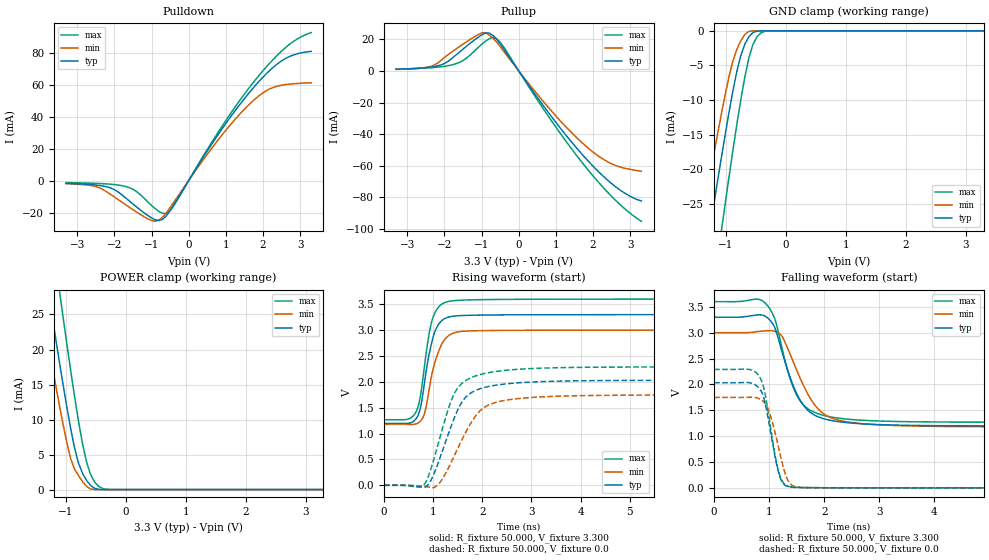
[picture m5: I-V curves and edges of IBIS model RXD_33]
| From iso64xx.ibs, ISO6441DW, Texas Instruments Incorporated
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|   RXD_33 Model
[Model]   RXD_33
Model_type   3-state
| Signals   RXD
Vmeas = 2.2V   |Reference voltage for timing measurements
Cref = 15pF   |Timing specification test load capacitance value
Vref = 0   |Timing specification test load voltage; GND
| variable   typ   min   max
C_comp   2.1pF   1.7pF   2.5pF
|   typ   min   max
[Temperature Range]   25.0   -40   125
[Voltage range]   3.3V   3.0V   3.6V
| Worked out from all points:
|   slope of the pulldown table from 0 to 0.495 V, typ, clamps not added: 27 ohm
|   slope of the pullup table from 0 to 0.495 V, typ, clamps not added: 29.8 ohm
|   GND clamp passes 1 mA (typ) near -0.63 V on its own axis
|   POWER clamp passes 1 mA (typ) near -0.62 V on its own axis
|   rising waveform, R_fixture 50.000, V_fixture 3.300: 20-80 % time 238ps typ, 270ps min, 219ps max; typ from 1.2 V to 3.3 V
|   rising waveform, R_fixture 50.000, V_fixture 0.0: 20-80 % time 505ps typ, 594ps min, 466ps max; typ from 0 V to 2.03 V
|   falling waveform, R_fixture 50.000, V_fixture 3.300: 20-80 % time 442ps typ, 514ps min, 392ps max; typ from 3.3 V to 1.2 V
|   falling waveform, R_fixture 50.000, V_fixture 0.0: 20-80 % time 217ps typ, 247ps min, 215ps max; typ from 2.03 V to 0 V
[Pulldown]
|Voltage   I(typ)   I(min)   I(max)
-3.3V     -1.746mA   -1.954mA   -1.317mA
-2.4V     -3.065mA   -4.531mA   -1.845mA
-1.7V     -10.79mA   -15.08mA   -3.688mA
-1.4V     -16.56mA   -19.75mA   -6.913mA
-900mV    -24.57mA   -25.5mA    -17.6mA
-600mV    -22.05mA   -20.21mA   -20.59mA
-400mV    -15.17mA   -13.54mA   -15.73mA
700mV     25.56mA    22.64mA    26.86mA
1.7V      56.99mA    49.23mA    60.23mA
2.1V      67.13mA    56.39mA    71.43mA
2.5V      74.94mA    59.69mA    81.03mA
3.3V      80.92mA    61.24mA    92.67mA
[Pullup]
|Voltage   I(typ)   I(min)   I(max)
-3.3V     1.146mA    992.8uA    1.173mA
-2.5V     2.119mA    2.237mA    1.881mA
-2.1V     3.82mA     6.606mA    2.666mA
-1.5V     13.89mA    17.02mA    6.669mA
-1V       22.84mA    24.1mA     16.9mA
-800mV    24.1mA     22.86mA    20.41mA
-600mV    20.3mA     18.51mA    20.5mA
-400mV    13.92mA    12.34mA    14.99mA
700mV     -23.25mA   -20.4mA    -25.37mA
1.7V      -52.69mA   -45.38mA   -57.86mA
2.5V      -71.39mA   -58.82mA   -79.5mA
3.3V      -82.38mA   -63.55mA   -95.26mA
[GND_clamp]
|Voltage   I(typ)   I(min)   I(max)
-3.3V     -145mA     -121.7mA   -175mA
-1.424V   -37.25mA   -28.36mA   -50.84mA
-1.29V    -29.79mA   -21.9mA    -42.24mA
-1.223V   -26.11mA   -18.72mA   -37.97mA
-1.089V   -18.87mA   -12.5mA    -29.55mA
-1.022V   -15.36mA   -9.534mA   -25.41mA
-821mV    -5.911mA   -2.691mA   -13.56mA
-754mV    -3.587mA   -1.433mA   -9.951mA
-620mV    -866.1uA   -93.64uA   -3.947mA
-486mV    -44.39uA   -245.8nA   -879.4uA
-352mV    -377.3nA   -292.5pA   -83.51uA
3.3V      0A         0A         0A
[POWER_clamp]
|Voltage   I(typ)   I(min)   I(max)
-3.3V     144.8mA    121.5mA    175.1mA
-1.457V   37.64mA    28.8mA     50.97mA
-1.39V    33.85mA    25.52mA    46.59mA
-1.256V   26.35mA    19.04mA    37.91mA
-1.122V   19.03mA    12.73mA    29.39mA
-1.055V   15.47mA    9.712mA    25.21mA
-921mV    8.813mA    4.477mA    17.12mA
-854mV    5.956mA    2.907mA    13.29mA
-720mV    2.301mA    1.133mA    6.51mA
-586mV    594.1uA    80.22uA    2.141mA
-318mV    345.9nA    220.3pA    41.12uA
3.3V      0A         0A         0A
[Ramp]
| variable   typ   min   max
dV/dt_r   1.219/0.505n   1.049/0.594n   1.374/0.467n
dV/dt_f   1.262/0.442n   1.093/0.514n   1.399/0.392n
R_load = 50.000
[Rising Waveform]
R_fixture= 50.000
V_fixture= 3.300
V_fixture_min= 3.000
V_fixture_max= 3.600
|time   V(typ)   V(min)   V(max)
0s        1.197V     1.178V     1.268V
469ps     1.196V     1.177V     1.274V
644ps     1.274V     1.185V     1.404V
733ps     1.462V     1.231V     1.675V
824ps     1.976V     1.388V     2.299V
913ps     2.502V     1.815V     2.896V
981ps     2.793V     2.169V     3.196V
1.17ns    3.178V     2.717V     3.499V
1.341ns   3.259V     2.911V     3.56V
15ns      3.3V       3V         3.6V
[Rising Waveform]
R_fixture= 50.000
V_fixture= 0.0
V_fixture_min= 0.0
V_fixture_max= 0.0
|time   V(typ)   V(min)   V(max)
0s        385.3nV    211.2nV    1.176uV
820ps     -34.98mV   -20.2mV    18.14mV
933ps     57.96mV    -40.03mV   254mV
1.105ns   437.4mV    19.91mV    808.4mV
1.454ns   1.354V     617.7mV    1.812V
1.634ns   1.672V     969.8mV    2.006V
1.864ns   1.834V     1.34V      2.115V
2.204ns   1.925V     1.581V     2.191V
4.104ns   2.023V     1.735V     2.282V
15ns      2.031V     1.748V     2.289V
[Falling Waveform]
R_fixture= 50.000
V_fixture= 3.300
V_fixture_min= 3.000
V_fixture_max= 3.600
|time   V(typ)   V(min)   V(max)
0s        3.3V       3V         3.6V
914ps     3.326V     3.033V     3.586V
1.105ns   3.091V     3.027V     3.26V
1.237ns   2.618V     2.927V     2.689V
1.388ns   2.113V     2.565V     2.084V
1.538ns   1.743V     2.18V      1.722V
1.864ns   1.385V     1.555V     1.442V
2.244ns   1.282V     1.314V     1.35V
4.338ns   1.201V     1.185V     1.272V
15ns      1.197V     1.178V     1.268V
[Falling Waveform]
R_fixture= 50.000
V_fixture= 0.0
V_fixture_min= 0.0
V_fixture_max= 0.0
|time   V(typ)   V(min)   V(max)
0s        2.031V     1.748V     2.289V
605ps     2.036V     1.75V      2.294V
817ps     1.927V     1.725V     2.162V
899ps     1.75V      1.664V     1.95V
986ps     1.321V     1.514V     1.442V
1.102ns   633.7mV    1.091V     661.1mV
1.172ns   292.6mV    774.7mV    312mV
1.294ns   47.58mV    266.2mV    59.06mV
1.404ns   13.21mV    60.12mV    17.7mV
15ns      723.6pV    692.4pV    123.1nV
